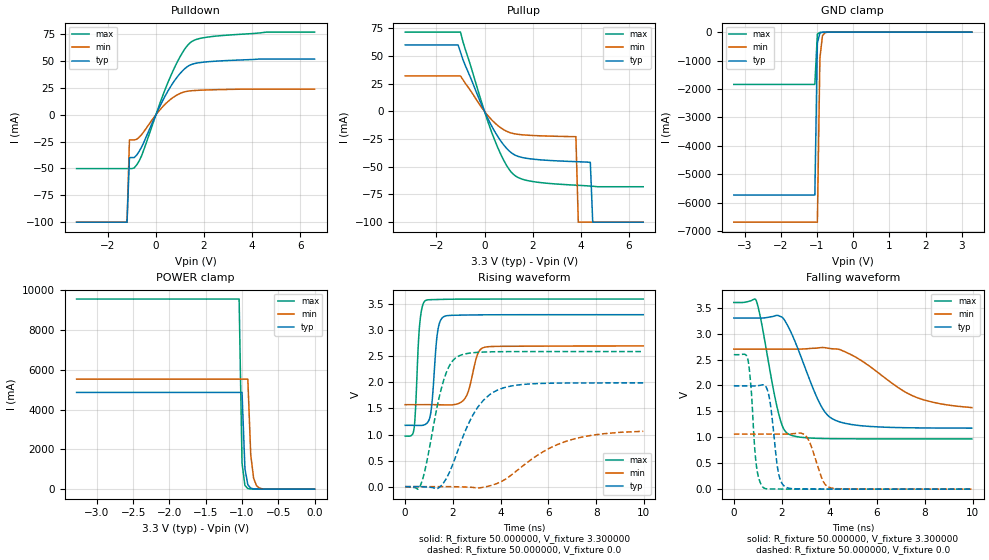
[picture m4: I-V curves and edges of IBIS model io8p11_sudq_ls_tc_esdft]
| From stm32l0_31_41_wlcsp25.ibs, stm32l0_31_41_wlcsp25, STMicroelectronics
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|   Model io8p11_sudq_ls_tc_esdft
[Model]  io8p11_sudq_ls_tc_esdft
Model_type I/O
Polarity   Non-Inverting
Enable   Active-Low
Vinl =   0.990000V
Vinh =   2.310000V
Vmeas =  1.650000V
Cref =   50.000000pF
Rref =   100.000000M
Vref =   0.0V
C_comp   2.248300pF   2.207300pF   2.311900pF
[Temperature Range]   25.000000   0.125000k   -40.000000
[Pullup Reference]   3.300000V   2.700000V   3.600000V
[Pulldown Reference]   0.0V   0.0V   0.0V
[POWER Clamp Reference]   3.300000V   2.700000V   3.600000V
[GND Clamp Reference]   0.0V   0.0V   0.0V
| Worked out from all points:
|   slope of the pulldown table from 0 to 0.495 V, typ, clamps not added: 22.6 ohm
|   slope of the pullup table from 0 to 0.495 V, typ, clamps not added: 23.9 ohm
|   GND clamp passes 1 mA (typ) near -0.64 V on its own axis
|   POWER clamp passes 1 mA (typ) near -0.63 V on its own axis
|   rising waveform, R_fixture 50.000000, V_fixture 3.300000: 20-80 % time 210ps typ, 365ps min, 166ps max; typ from 1.18 V to 3.3 V
|   rising waveform, R_fixture 50.000000, V_fixture 0.0: 20-80 % time 1.19ns typ, 2.2ns min, 713ps max; typ from 0 V to 1.99 V
|   falling waveform, R_fixture 50.000000, V_fixture 3.300000: 20-80 % time 1.12ns typ, 2.14ns min, 643ps max; typ from 3.3 V to 1.18 V
|   falling waveform, R_fixture 50.000000, V_fixture 0.0: 20-80 % time 291ps typ, 461ps min, 230ps max; typ from 1.99 V to 0 V
[Pulldown]
|Voltage   I(typ)   I(min)   I(max)
-3.3V     -100mA     -100mA     -50.11mA
-1.2V     -100mA     -100mA     -50.11mA
-1.1V     -39.8mA    -23.38mA   -50.11mA
-900mV    -39.8mA    -23.38mA   -49.43mA
-600mV    -30.26mA   -18.59mA   -38.38mA
500mV     22.11mA    12.28mA    30.06mA
900mV     35.58mA    18.71mA    49.62mA
1.3V      44.73mA    21.88mA    64.23mA
1.7V      48.13mA    22.72mA    70.3mA
2.4V      49.79mA    23.3mA     73.03mA
4.6V      51.9mA     23.82mA    77mA
6.6V      51.9mA     23.82mA    77mA
[Pullup]
|Voltage   I(typ)   I(min)   I(max)
-3.3V     60mA       32mA       71.6mA
-1.1V     60mA       32mA       71.6mA
-1V       53.5mA     32mA       71.6mA
-100mV    4.893mA    2.926mA    6.861mA
400mV     -17.21mA   -9.813mA   -24.69mA
900mV     -32.92mA   -17.72mA   -48.15mA
1.3V      -39.75mA   -20.41mA   -58.47mA
3.8V      -45.36mA   -22.8mA    -66.6mA
3.9V      -45.44mA   -100mA     -66.72mA
4.4V      -46mA      -100mA     -67.4mA
4.5V      -100mA     -100mA     -67.56mA
6.6V      -100mA     -100mA     -68mA
[GND_clamp]
|Voltage   I(typ)   I(min)   I(max)
-3.3V     -5.732A    -6.688A    -1.842A
-1.06V    -5.732A    -6.688A    -1.842A
-990mV    -389.4mA   -6.688A    -68.34mA
-920mV    -32.57mA   -918.2mA   -10.72mA
-850mV    -6.763mA   -131mA     -6.509mA
-780mV    -3.471mA   -21mA      -4.208mA
3.28V     0A         0A         0A
[POWER_clamp]
|Voltage   I(typ)   I(min)   I(max)
-3.28V    4.87A      5.538A     9.569A
-1.04V    4.87A      5.538A     9.569A
-1V       4.87A      5.538A     1.315A
-960mV    1.032A     5.538A     186.5mA
-920mV    222.2mA    5.538A     31.64mA
-880mV    50.73mA    1.734A     9.582mA
-840mV    13.93mA    544.8mA    5.668mA
-800mV    5.556mA    172.7mA    4.276mA
-760mV    3.231mA    55.84mA    3.297mA
-680mV    1.597mA    6.983mA    1.741mA
0V        0A         0A         0A
[Ramp]
| variable   typ   min   max
dV/dt_r  1.19466/1.19320n   0.60726/2.06111n   1.55562/0.71176n
dV/dt_f  1.27218/1.11984n   0.59286/1.92693n   1.57784/0.64216n
R_load = 50.000000
[Rising Waveform]
R_fixture= 50.000000
V_fixture= 3.300000
V_fixture_min= 2.700000
V_fixture_max= 3.600000
|time   V(typ)   V(min)   V(max)
0s        1.177V     1.573V     969.3mV
360.4ps   1.176V     1.573V     1.081V
600.6ps   1.173V     1.573V     3.08V
860.9ps   1.199V     1.573V     3.573V
1.081ns   1.443V     1.573V     3.589V
1.381ns   3.034V     1.572V     3.592V
1.642ns   3.268V     1.569V     3.595V
2.523ns   3.293V     1.705V     3.599V
3.323ns   3.298V     2.675V     3.6V
9.97ns    3.3V       2.7V       3.6V
[Rising Waveform]
R_fixture= 50.000000
V_fixture= 0.0
V_fixture_min= 0.0
V_fixture_max= 0.0
|time   V(typ)   V(min)   V(max)
0s        -1.608uV   12.65uV    -132.9uV
640.6ps   -938uV     -6.166uV   24.98mV
840.8ps   -5.316mV   6.654uV    341.2mV
1.562ns   47.19mV    182.2uV    1.962V
1.862ns   284.7mV    -362.7uV   2.328V
2.182ns   662.4mV    -2.668mV   2.492V
3.063ns   1.538V     -25.78mV   2.578V
4.024ns   1.881V     96.92mV    2.59V
6.687ns   1.988V     861.9mV    2.593V
9.97ns    1.992V     1.062V     2.593V
[Falling Waveform]
R_fixture= 50.000000
V_fixture= 3.300000
V_fixture_min= 2.700000
V_fixture_max= 3.600000
|time   V(typ)   V(min)   V(max)
0s        3.3V       2.7V       3.6V
940.9ps   3.3V       2.7V       3.636V
1.822ns   3.352V     2.7V       1.563V
2.062ns   3.3V       2.7V       1.188V
2.282ns   3.131V     2.7V       1.066V
3.564ns   1.687V     2.726V     978.7mV
4.124ns   1.358V     2.707V     973.8mV
5.085ns   1.237V     2.552V     970.7mV
7.528ns   1.183V     1.793V     969.4mV
9.97ns    1.177V     1.573V     969.3mV
[Falling Waveform]
R_fixture= 50.000000
V_fixture= 0.0
V_fixture_min= 0.0
V_fixture_max= 0.0
|time   V(typ)   V(min)   V(max)
0s        1.992V     1.062V     2.593V
600.6ps   1.992V     1.062V     2.476V
940.9ps   1.993V     1.062V     472.1mV
1.261ns   2.009V     1.062V     22.29mV
1.502ns   1.728V     1.062V     4.269mV
1.882ns   287.5mV    1.062V     2.683mV
2.182ns   38.3mV     1.062V     2.081mV
3.043ns   3.071mV    1.011V     879.9uV
4.084ns   1.478mV    21.96mV    206.7uV
9.97ns    -1.608uV   12.65uV    -132.9uV
